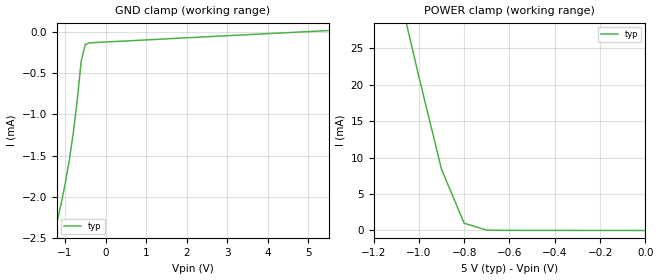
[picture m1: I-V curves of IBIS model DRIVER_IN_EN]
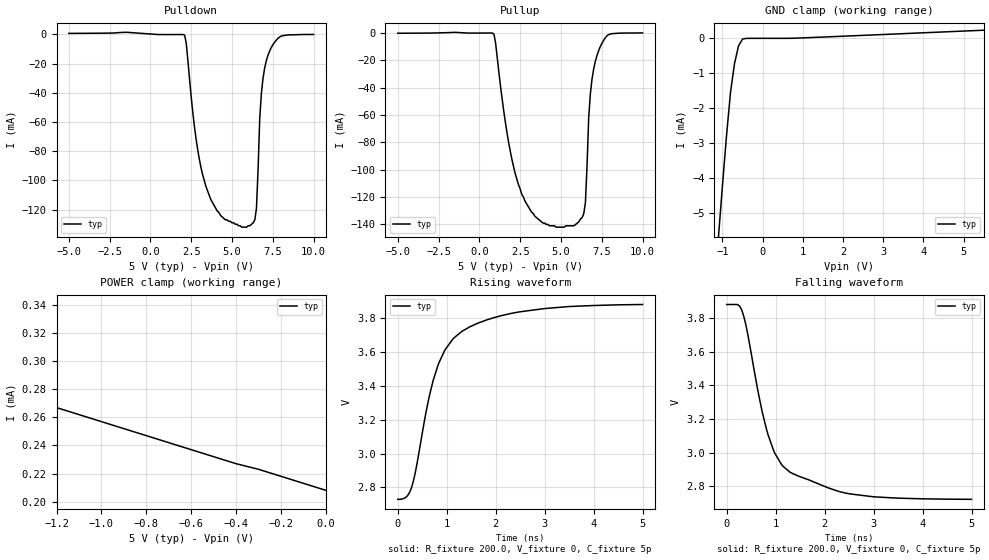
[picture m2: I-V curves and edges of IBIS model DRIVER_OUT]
|   Texas Instruments Incorporated
|   Data Transmissions Products
|   IBIS Model for TB5D2H
|   16DW SOIC Package
[IBIS Ver]   3.2
[Comment char]   |_char
[File name]   tb5d2h.ibs
[File Rev]   1.0
[Date]   14Apr03
[Source]   File originated at Texas Instruments Incorporated.
   Data Transmission Products Group. All data based on
   simulation.
[Notes]
[Disclaimer]
(C) Copyright Texas Instruments Incorporated 2003
   All rights reserved
  Texas Instruments Incorporated hereby grants the user of this IBIS
model a non-exclusive, nontransferable license to use this IBIS model
under the following terms.  Before using this IBIS model, the user
should read this license.  If the user does not accept these terms,
the IBIS model should be returned to Texas Instruments within 30 days.
  The user is granted this license only to use the IBIS model and
is not granted rights to sell, load, rent, lease or license the IBIS
model in whole or in part, or in modified form to anyone other than
user.  User may modify the IBIS model to suit its specific applications
but rights to derivative works and such modifications shall belong to
Texas Instruments.
  This IBIS model is provided on an "AS IS" basis and Texas Instruments
makes absolutely no warranty with respect to the information contained
herein.  TEXAS INSTRUMENTS DISCLAIMS AND CUSTOMER WAIVES ALL WARRANTIES,
EXPRESS OR IMPLIED, INCLUDING WARRANTIES OF MERCHANTABILITY OR FITNESS
FOR A PARTICULAR PURPOSE. The entire risk as to quality and performance
is with the Customer. ACCORDINGLY, IN NO EVENT SHALL THE COMPANY BE LIABLE
FOR ANY DAMAGES, WHETHER IN CONTRACT OR TORT,INCLUDING ANY LOST PROFITS
OR OTHER INCIDENTAL, CONSEQUENTIAL, EXEMPLARY, OR PUNITIVE DAMAGES ARISING
OUT OF THE USE OR APPLICATION OF THE IBIS model provided in this package.
Further, Texas Instruments reserves the right to discontinue or make changes
without notice to any product herein to improve reliability, function, or
design. Texas Instruments does not convey any license under patent rights
or any other intellectual property rights, including those of third parties.
Contact Texas Instruments at ATTN:DATA TRANSMISSIONS
[Copyright]   Copyright 2003, Texas Instruments, All Rights Reserved
[Component]   TB5D2H
[Manufacturer]  Texas Instruments
[Package]
|   typ   min   max
R_pkg   0.046   0.034   0.057
L_pkg   4.858nH   3.987nH   6.214nH
C_pkg   0.715pF   0.502pF   1.046pF
[Pin]   signal_name   model_name   R_pin   L_pin   C_pin
1   AI   DRIVER_IN_EN   0.057   6.214nH   1.026pF
2   AO   DRIVER_OUT   0.055   5.236nH   0.818pF
3   AO(-)   DRIVER_OUT   0.034   3.987nH   0.723pF
4   E1   DRIVER_IN_EN   0.036   3.996nH   0.726pF
5   BO(-)   DRIVER_OUT   0.036   3.996nH   0.726pF
6   BO   DRIVER_OUT   0.034   3.987nH   0.704pF
7   BI   DRIVER_IN_EN   0.055   5.236nH   0.818pF
8   GND   GND   0.057   6.214nH   1.046pF
9   CI   DRIVER_IN_EN   0.057   6.214nH   0.827pF
10   CO   DRIVER_OUT   0.055   5.236nH   0.597pF
11   CO(-)   DRIVER_OUT   0.034   3.987nH   0.502pF
12   E2   DRIVER_IN_EN   0.036   3.996nH   0.505pF
13   DO(-)   DRIVER_OUT   0.036   3.996nH   0.505pF
14   DO   DRIVER_OUT   0.034   3.987nH   0.502pF
15   DI   DRIVER_IN_EN   0.055   5.236nH   0.597pF
16   VCC   POWER   0.057   6.214nH   0.827pF
[Diff_pin]   inv_pin   vdiff   tdelay_typ   tdelay_min   tdelay_max
| The 'AO(+) (or 'xO(+)')' and inv_pins, 'AO(-) (or 'xO(-)')', pins
| are Diff_pins
   2   3   0   0   0   0
   6   5   0   0   0   0
   10   11   0   0   0   0
   14   13   0   0   0   0
| Models and submodels in the file (2): DRIVER_IN_EN (Input), DRIVER_OUT (Output_ECL)
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|   Driver Input Model
[Model]   DRIVER_IN_EN
Model_type   Input
|Signals   AI,BI,CI,DI,E1,E2
Vinh = 2.4
Vinl = 0.4
|   typ   min   max
C_comp   979fF   NA   NA
|   typ   min   max
[Temperature Range]   25.0   NA   NA
[Voltage range]   5.0V   NA   NA
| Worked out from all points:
|   GND clamp passes 1 mA (typ) near -0.74 V on its own axis
|   POWER clamp passes 1 mA (typ) near -0.80 V on its own axis
[GND_clamp]
| Voltage   I(typ)   I(min)   I(max)
-5.5V     -10.4mA    NA         NA
-1.3V     -2.52mA    NA         NA
-1.2V     -2.31mA    NA         NA
-1.1V     -2.09mA    NA         NA
-1V       -1.85mA    NA         NA
-900mV    -1.57mA    NA         NA
-800mV    -1.24mA    NA         NA
-700mV    -830uA     NA         NA
-600mV    -351uA     NA         NA
-500mV    -156uA     NA         NA
-300mV    -132uA     NA         NA
5.5V      13.7uA     NA         NA
[Power_clamp]
| Note that the[POWER_clamp]voltage table is referenced to Vcc
| and is calculated using Vtable=Vcc - Vmeasured.
|   Voltage   I(typ)   I(min)   I(max)
-5V       163mA      NA         NA
-1.1V     34.4mA     NA         NA
-1V       21.1mA     NA         NA
-900mV    8.39mA     NA         NA
-800mV    993uA      NA         NA
-700mV    43.9uA     NA         NA
0V        1.12uA     NA         NA
|   Driver Output Model
[Model]   DRIVER_OUT
|Model_type   3-state_ECL
Model_type   Output_ECL
| Signals   O(+),O(-)
Vmeas = 3.2V   |Reference voltage for timing measurements
Cref = 5pF   |Timing specification test load capacitance value
Rref = 200   |Note: 200 Ohm load; single ended configuration
| variable   typ   min   max
C_comp   553fF   NA   NA
|   typ   min   max
[Temperature Range]   25.0   NA   NA
[Voltage range]   5.0V   NA   NA
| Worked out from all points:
|   GND clamp passes 1 mA (typ) near -0.73 V on its own axis
|   POWER clamp passes 1 mA (typ) near -1.95 V on its own axis
|   rising waveform, R_fixture 200.0, V_fixture 0, C_fixture 5p: 20-80 % time 654ps typ, NA min, NA max; typ from 2.73 V to 3.88 V
|   falling waveform, R_fixture 200.0, V_fixture 0, C_fixture 5p: 20-80 % time 604ps typ, NA min, NA max; typ from 3.88 V to 2.72 V
[Pulldown]
|   Voltage   I(typ)   I(min)   I(max)
-5V       650uA      NA         NA
2.1V      -573uA     NA         NA
2.8V      -71.6mA    NA         NA
3.4V      -104mA     NA         NA
5.6V      -132mA     NA         NA
6.4V      -127mA     NA         NA
6.5V      -119mA     NA         NA
6.7V      -57.6mA    NA         NA
6.8V      -40.6mA    NA         NA
7.2V      -14.5mA    NA         NA
8V        -1.3mA     NA         NA
10V       -100uA     NA         NA
[Pullup]
|   Voltage   I(typ)   I(min)   I(max)
| Note that the[Pullup]voltage table is referenced to Vcc
| and is calculated using Vtable=Vcc - Vmeasured.
-5V       -351uA     NA         NA
900mV     -1.15mA    NA         NA
1.8V      -80.4mA    NA         NA
2.6V      -118mA     NA         NA
3.9V      -139mA     NA         NA
5.2V      -142mA     NA         NA
6.4V      -132mA     NA         NA
6.5V      -124mA     NA         NA
6.7V      -62.2mA    NA         NA
6.8V      -44.8mA    NA         NA
7.4V      -10.4mA    NA         NA
10V       -100uA     NA         NA
[GND_clamp]
|   Voltage   I(typ)   I(min)   I(max)
| Outputs in High Impedance (off)
-5.5V     -173mA     NA         NA
-1.1V     -5.68mA    NA         NA
-1V       -4.2mA     NA         NA
-900mV    -2.79mA    NA         NA
-800mV    -1.54mA    NA         NA
-700mV    -719uA     NA         NA
-600mV    -212uA     NA         NA
-500mV    -19.1uA    NA         NA
900mV     8.68uA     NA         NA
5.5V      232uA      NA         NA
[Power_clamp]
| Note that the[POWER_clamp]voltage table is referenced to Vcc
| and is calculated using Vtable=Vcc - Vmeasured.
|   Voltage   I(typ)   I(min)   I(max)
-5V       4.97mA     NA         NA
-1.5V     350uA      NA         NA
-1.4V     292uA      NA         NA
-1.3V     273uA      NA         NA
-1.2V     267uA      NA         NA
-400mV    227uA      NA         NA
-300mV    223uA      NA         NA
0V        208uA      NA         NA
[Ramp]
|   typ   min   max
dV/dt_r   0.694/659ps   NA   NA
dV/dt_f   0.694/605ps   NA   NA
R_load = 200ohm
[Rising Waveform]
R_fixture = 200.0
V_fixture = 0
C_fixture = 5p
|   V(typ)   V(min)   V(max)
0s        2.73V      NA         NA
175ps     2.744V     NA         NA
300ps     2.817V     NA         NA
625ps     3.312V     NA         NA
825ps     3.524V     NA         NA
975ps     3.617V     NA         NA
1.3ns     3.72V      NA         NA
1.825ns   3.791V     NA         NA
2.5ns     3.838V     NA         NA
5ns       3.881V     NA         NA
[Falling Waveform]
R_fixture = 200.0
V_fixture = 0
C_fixture = 5p
|   V(typ)   V(min)   V(max)
0s        3.882V     NA         NA
225ps     3.881V     NA         NA
300ps     3.854V     NA         NA
400ps     3.749V     NA         NA
650ps     3.35V      NA         NA
825ps     3.126V     NA         NA
1ns       2.988V     NA         NA
1.3ns     2.882V     NA         NA
2.5ns     2.755V     NA         NA
5ns       2.722V     NA         NA
